(* Logix 5000 DataType export ToloInput; software revision 20.01 *)

TYPE DriveFaults :
STRUCT
   Positive_Limit : BOOL;   // Positive Limit
   Negative_Limit : BOOL;   // Negative Limit
   E_Stop : BOOL;   // E Stop
   Position_Error : BOOL;   // Position Error
   Feedback_Error : BOOL;   // Feedback Error
   Over_Current : BOOL;   // Overcurrent
   Motor_Over_Temperature : BOOL;   // Motor Over Temperature
   Drive_Over_Temperature : BOOL;   // Drive Over Temperature
   Drive_Over_Voltage : BOOL;   // Drive Over Voltage
   Drive_Under_Voltage : BOOL;   // Drive Under Voltage
   Flash_Error : BOOL;   // Flash Error
   I2T_Limit : BOOL;   // I2T Limit Fault
   Short_Circuit : BOOL;   // Short Circuit Fault
   Watchdog_Reset : BOOL;   // Watchdog Reset
END_STRUCT
END_TYPE

TYPE DriveStatus :
STRUCT
   Drive_Enable : BOOL;   // Drive Enable Input
   Drive_Homed : BOOL;   // Drive Home Input
   Drive_InMotion : BOOL;   // Drive In Motion Input
   Drive_EStop : BOOL;   // Drive E-Stop Input
   rsved_bit00 : BOOL;
   rsved_bit01 : BOOL;
   rsved_bit02 : BOOL;
   rsved_bit03 : BOOL;
   rsved_bit04 : BOOL;
   rsved_bit05 : BOOL;
   rsved_bit06 : BOOL;
   rsved_bit07 : BOOL;
   rsved_bit08 : BOOL;
   Drive_EthAvail : BOOL;   // Drive Ethernet Online
   rsved_bit09 : BOOL;
   rsved_bit10 : BOOL;
   rsved_bit11 : BOOL;
   rsved_bit12 : BOOL;
   rsved_bit13 : BOOL;
   rsved_bit14 : BOOL;
   Drive_BrakeOff : BOOL;   // Brake Output (0 - Enabled; 1- Not Enabled)
   rsved_bit15 : BOOL;
   rsved_bit16 : BOOL;
   rsved_bit17 : BOOL;
   rsrved_bit18 : BOOL;
   rsrved_bit19 : BOOL;
   rsrved_bit20 : BOOL;
   rsrved_bit21 : BOOL;
   rsrved_bit22 : BOOL;
   rsrved_bit23 : BOOL;
   rsrved_bit24 : BOOL;
   Drive_Control : BOOL;
END_STRUCT
END_TYPE

TYPE ToloInput :
STRUCT
   Current_Position : REAL;   // Actuator Current Position
   DriveStatus : DriveStatus;
   DriveFaults : DriveFaults;
   Digital_Input : DINT;   // Digital Input Status
   Digital_Output : DINT;   // Digital Output Status
   Analog_Input : REAL;
   Analog_Output : REAL;
END_STRUCT
END_TYPE
